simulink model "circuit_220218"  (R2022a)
settings: Solver=VariableStepAuto  StartTime=-D+0.1e-6  StopTime=34e-6  FixedStep=1e-3  MaxStep=0.1e-6  RelTol=1e-3
model workspace (MATLAB code in the model file):
  sGeo = CreateGeometry()
  sConst = CreateConstants()
libraries: fl_lib x7, ee_lib x3, nesl_utility x3

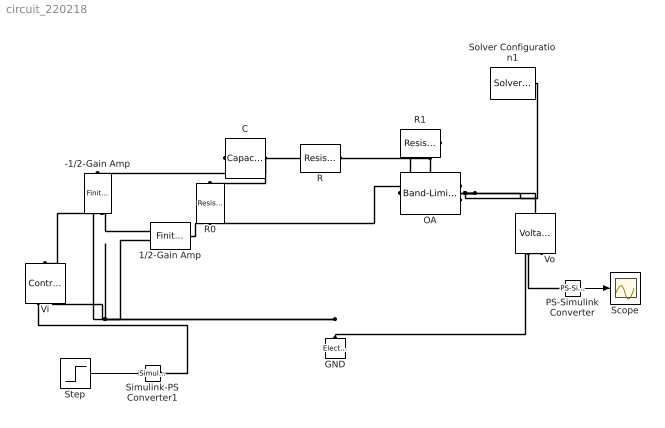
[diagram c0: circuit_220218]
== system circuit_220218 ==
  -1/2-Gain Amp : ee_lib/Integrated Circuits/Finite-Gain Op-Amp  A=0.5  Rin=1e6 Ohm  Rout=0 Ohm  Vmin=-15 V  Vmax=15 V  noise_mode=0  v_noise=30e-9 V/Hz^0.50000  noise_prm=1  i_noise=0.5e-12 A/Hz^0.50000  ip_noise=0.5e-12 A/Hz^0.50000  in_noise=0.5e-12 A/Hz^0.50000  sample_time=1e-3 s  repeatability=1  auto_seed_v=1698724916  auto_seed_ip=1578128389  auto_seed_in=4243350392  user_seed_v=0  user_seed_ip=0  user_seed_in=0
  1/2-Gain Amp : ee_lib/Integrated Circuits/Finite-Gain Op-Amp  A=0.5  Rin=1e6 Ohm  Rout=0 Ohm  Vmin=-15 V  Vmax=15 V  noise_mode=0  v_noise=30e-9 V/Hz^0.50000  noise_prm=1  i_noise=0.5e-12 A/Hz^0.50000  ip_noise=0.5e-12 A/Hz^0.50000  in_noise=0.5e-12 A/Hz^0.50000  sample_time=1e-3 s  repeatability=1  auto_seed_v=1366117752  auto_seed_ip=512022555  auto_seed_in=4036536839  user_seed_v=0  user_seed_ip=0  user_seed_in=0
  C : fl_lib/Electrical/Electrical Elements/Capacitor  c=15 nF  r=0 Ohm  g=0 1/Ohm  i_specify=off  i_priority=None  i=0 A  i_nominal_specify=off  i_nominal_unit=A  i_nominal_value=1  v_specify=off  v_priority=None  v=0 V  v_nominal_specify=off  v_nominal_unit=V  v_nominal_value=1  vc_specify=off  vc_priority=High  vc=0 V  vc_nominal_specify=off  vc_nominal_unit=V  vc_nominal_value=1
  GND : fl_lib/Electrical/Electrical Elements/Electrical Reference
  OA : ee_lib/Integrated Circuits/Band-Limited Op-Amp  A=100000  Rin=1e8 Ohm  Rout=0 Ohm  Vmin=-15 V  Vmax=15 V  Vdotmax=1000000 V/s  f=20 Hz  V0=0 V
  PS-Simulink Converter : nesl_utility/PS-Simulink Converter  PhysicalDomain=network_engine_domain  SubClassName=ps_output  LeftPortType=input  RightPortType=output  PseudoPeriodic=off  Frequencies=[]  VectorFormat=1-D array  Unit=inherit  AffineConversion=off
  R : fl_lib/Electrical/Electrical Elements/Resistor  R=10 kOhm  i_specify=off  i_priority=None  i=0 A  i_nominal_specify=off  i_nominal_unit=A  i_nominal_value=1  v_specify=off  v_priority=None  v=0 V  v_nominal_specify=off  v_nominal_unit=V  v_nominal_value=1
  R0 : fl_lib/Electrical/Electrical Elements/Resistor  R=10 kOhm  i_specify=off  i_priority=None  i=0 A  i_nominal_specify=off  i_nominal_unit=A  i_nominal_value=1  v_specify=off  v_priority=None  v=0 V  v_nominal_specify=off  v_nominal_unit=V  v_nominal_value=1
  R1 : fl_lib/Electrical/Electrical Elements/Resistor  R=100 kOhm  i_specify=off  i_priority=None  i=0 A  i_nominal_specify=off  i_nominal_unit=A  i_nominal_value=1  v_specify=off  v_priority=None  v=0 V  v_nominal_specify=off  v_nominal_unit=V  v_nominal_value=1
  Scope : Scope
  Simulink-PS Converter1 : nesl_utility/Simulink-PS Converter  PhysicalDomain=network_engine_domain  SubClassName=ps_input  LeftPortType=input  RightPortType=output  PseudoPeriodic=off  Frequencies=[]  NoiseDistribution=none  NoiseParameters=[]  Unit=1  AffineConversion=off  FilteringAndDerivatives=provide  SimscapeFilterOrder=1  InputFilterTimeConstant=0.001  UdotUserProvided=0
  Solver Configuration1 : nesl_utility/Solver Configuration  PhysicalDomain=network_engine_domain  SubClassName=solver  LeftPortType=input  RightPortType=generic  Tones=[]  Harmonics=[]  SimulateNoise=off  Profile=off  UseLocalSampling=off  EnableSwitchedLinearOptims=on  FrequencyDomain=off  UseCCode=off  RelTol=0.001  AbsTol=1e-06  MinStep=1e-09  ToWorkspace=off  RevertToSquareIcSolve=off  NumHomotopyIterations=100  PhasorMode=off  PhasorModeNumHarmonics=1  IndexReductionMethod=DerivativeReplacement  DoDC=off  ResidualTolerance=1e-09  UseLocalSolver=off  LocalSolverChoice=NE_BACKWARD_EULER_ADVANCER  LocalSolverSampleTime=0.001  DoFixedCost=off  MaxNonlinIter=3  MaxModeIter=2  ComputeImpulses=off  ImpulseIterations=2  LinearAlgebra=Sparse  LinearAlgebraNumThread=0  EquationFormulation=NE_TIME_EF  DelaysMemoryBudget=1024  AutomaticFiltering=on  FilteringTimeConstant=0.001  PartitionStorageMethod=AS_NEEDED  PartitionMemoryBudget=1024  PartitionMethod=FAST
  Step : Step  SampleTime=0
  Vi : fl_lib/Electrical/Electrical Sources/Controlled Voltage Source
  Vo : fl_lib/Electrical/Electrical Sensors/Voltage Sensor
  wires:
  Step/1 -> Simulink-PS Converter1/1
  PS-Simulink Converter/1 -> Scope/1
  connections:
  -1/2-Gain Amp/LConn2 -- 1/2-Gain Amp/LConn1 -- Vi/LConn1
  Vo/RConn1 -- PS-Simulink Converter/LConn1
  OA/RConn1 -- R1/LConn1 -- Solver Configuration1/RConn1 -- Vo/LConn1
  GND/LConn1 -- Vi/RConn2 -- 1/2-Gain Amp/LConn2 -- -1/2-Gain Amp/LConn1 -- Vo/RConn2
  R1/RConn1 -- R/LConn1 -- OA/LConn2
  Vi/RConn1 -- Simulink-PS Converter1/RConn1
  R/RConn1 -- C/LConn1
  C/RConn1 -- R0/LConn1 -- -1/2-Gain Amp/RConn1
  R0/RConn1 -- OA/LConn1 -- 1/2-Gain Amp/RConn1
